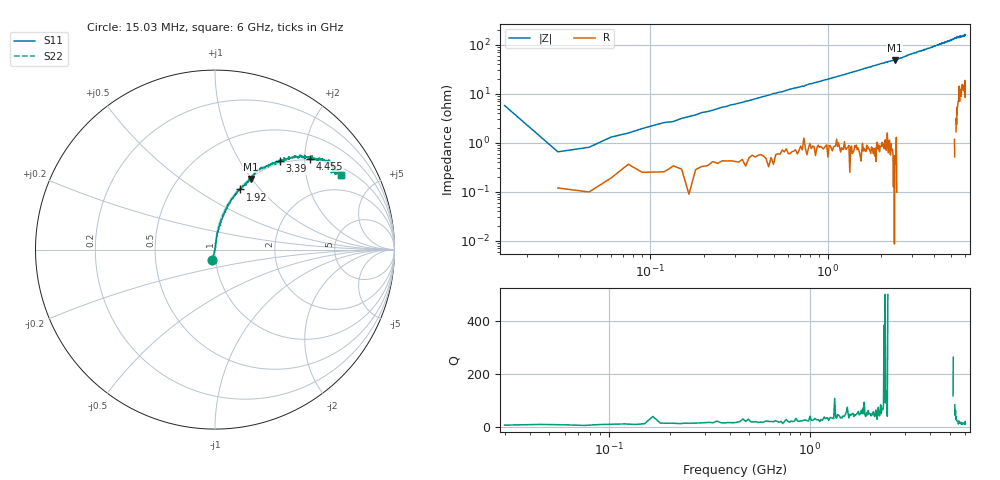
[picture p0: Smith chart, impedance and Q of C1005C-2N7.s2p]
!	Network	Analyzer	HP8753E.07.74:	Oct	30	2002	Serial	No.	JP38451487
!	Hewlett-Packard
!	7	Sep	2009	8:21:07
!	Frequency	S11	S21	S12	S22
#	HZ	S	RI	R	50
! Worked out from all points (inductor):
!   400 points, 15.03 MHz to 6 GHz, reference 50 ohm
!   read as one part in series: L = 3.27 nH near 45.03 MHz
!   highest Q = 91.5 at 2.4 GHz (marker M1), where L = 3.27 nH
!   S11 on the Smith chart (normalised r, x): 15.03 MHz: 0.96, -0.11; 1.92 GHz: 1.02, +0.78; 3.39 GHz: 0.96, +1.52; 4.455 GHz: 0.97, +2.13; 6 GHz: 1.29, +3.18
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1.502992e7  -0.0147 -0.057  1.01 0.057  1.01 0.057  -0.0147 -0.057
3.002985e7  0.00148 0.00643  0.999 -0.00643  0.999 -0.00643  0.00148 0.00643
4.502978e7  0.00111 0.00803  0.999 -0.00803  0.999 -0.00803  0.00111 0.00803
6.00297e7  0.00216 0.0129  0.998 -0.0129  0.998 -0.0129  0.00216 0.0129
1.050295e8  0.00307 0.0226  0.997 -0.0226  0.997 -0.0226  0.00307 0.0226
1.95029e8  0.00494 0.041  0.995 -0.041  0.995 -0.041  0.00494 0.041
2.850286e8  0.00751 0.0587  0.992 -0.0587  0.992 -0.0587  0.00751 0.0587
6.150269e8  0.0209 0.121  0.979 -0.121  0.979 -0.121  0.0209 0.121
1.020025e9  0.0469 0.191  0.953 -0.191  0.953 -0.191  0.0469 0.191
1.92002e9  0.139 0.335  0.861 -0.335  0.861 -0.335  0.139 0.335
2.01002e9  0.151 0.348  0.849 -0.348  0.849 -0.348  0.151 0.348
2.400018e9  0.198 0.393  0.802 -0.393  0.802 -0.393  0.198 0.393
3.015015e9  0.299 0.474  0.701 -0.474  0.701 -0.474  0.299 0.474
3.390013e9  0.363 0.494  0.637 -0.494  0.637 -0.494  0.363 0.494
4.00501e9  0.474 0.526  0.526 -0.526  0.526 -0.526  0.474 0.526
4.455008e9  0.531 0.507  0.469 -0.507  0.469 -0.507  0.531 0.507
5.010005e9  0.611 0.495  0.389 -0.495  0.389 -0.495  0.611 0.495
5.355003e9  0.673 0.461  0.327 -0.461  0.327 -0.461  0.673 0.461
5.535002e9  0.647 0.429  0.353 -0.429  0.353 -0.429  0.647 0.429
5.565002e9  0.687 0.441  0.313 -0.441  0.313 -0.441  0.687 0.441
5.595002e9  0.656 0.438  0.344 -0.438  0.344 -0.438  0.656 0.438
6e9  0.702 0.414  0.298 -0.414  0.298 -0.414  0.702 0.414
